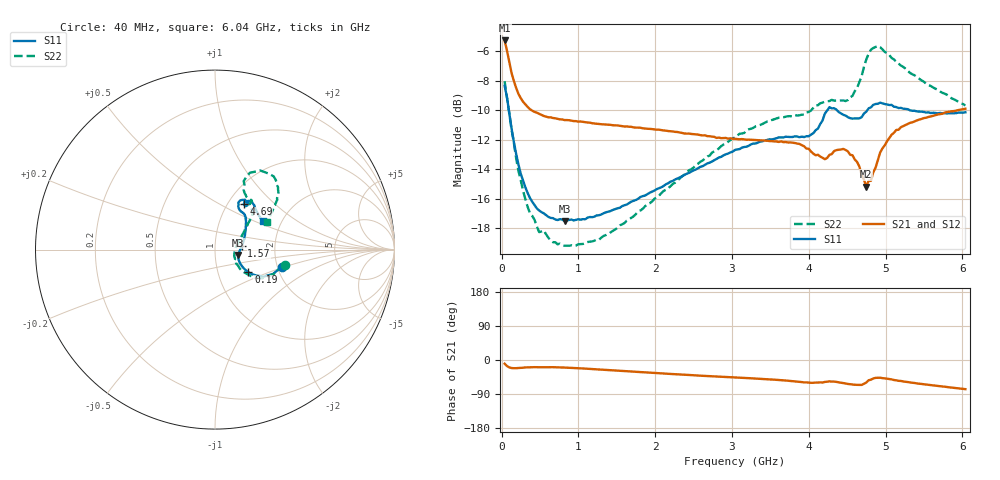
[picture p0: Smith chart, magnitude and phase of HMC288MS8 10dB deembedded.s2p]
!Hittite Microwave Corporation
!12 Elizabeth Drive
!Chelmsford, MA 01824
!Tel: 978-250-3343
!Fax: 978-250-3373
!Device: HMC288MS8, 0.7-3.7 GHz GaAs IC 3-bit Digital Attenuator in 8-lead Grounded Base surface Mount Plastic Package
!Misc:  10dB state, room
# GHZ S DB R 50.0
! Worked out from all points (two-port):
!   201 points, 40 MHz to 6.04 GHz, reference 50 ohm
!   highest |S21| = -5.26 dB at 40 MHz (marker M1); lowest = -15.2 dB at 4.75 GHz (marker M2)
!   |S21| within 3 dB of the highest: start of sweep to 176.5 MHz
!   lowest |S11| = -17.5 dB at 820 MHz (marker M3), VSWR 1.31, Z = 64.8 - j3.89 ohm
!   |S11| at or under -10 dB: 95.9 MHz to 4.242 GHz (4.146 GHz wide, 191 % of centre); 4.369 GHz to 4.762 GHz (392.4 MHz wide, 8.59 % of centre); 5.319 GHz to end of sweep
!   |S22| runs from -19.2 to -5.6 dB; largest |S21 - S12| = 0.0038
!   S11 on the Smith chart (normalised r, x): 40 MHz: 2.11, -0.47; 190 MHz: 1.40, -0.37; 1.57 GHz: 1.35, +0.05; 4.69 GHz: 1.18, +0.66; 6.04 GHz: 1.60, +0.57
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0.04  -8.33 -14.4  -5.26 -9.8  -5.32 -9.7  -8.02 -12.5
0.1  -10.14 -28.8  -6.70 -19.4  -6.74 -19.3  -10.22 -31.1
0.19  -12.94 -34.2  -8.48 -21.6  -8.49 -21.5  -13.25 -37.5
0.34  -15.61 -29.8  -9.77 -19.4  -9.76 -19.7  -16.54 -34.1
0.49  -16.79 -23.9  -10.24 -19.0  -10.22 -18.8  -18.25 -28.4
0.82  -17.49 -12.8  -10.66 -20.0  -10.63 -20.2  -19.18 -12.3
1.06  -17.38 -6.1  -10.78 -22.5  -10.77 -22.5  -19.06 -2.8
1.57  -16.50 7.3  -11.06 -28.8  -11.06 -28.9  -17.73 14.0
2.05  -15.28 20.1  -11.31 -34.9  -11.30 -35.0  -15.78 25.9
3.04  -12.69 41.6  -11.93 -46.0  -11.89 -46.1  -11.85 40.3
3.82  -11.76 52.6  -12.21 -56.2  -12.21 -56.2  -10.32 46.9
4.06  -11.55 60.0  -12.94 -60.2  -12.93 -60.2  -9.83 52.8
4.18  -10.69 63.6  -13.22 -59.4  -13.22 -59.6  -9.47 53.0
4.27  -9.79 59.0  -13.01 -56.4  -12.98 -56.6  -9.37 53.0
4.51  -10.46 54.4  -12.78 -63.2  -12.76 -63.5  -9.30 59.3
4.69  -10.46 57.7  -14.40 -65.8  -14.35 -66.0  -7.66 67.3
4.75  -10.09 58.4  -15.17 -59.4  -15.09 -59.1  -6.55 65.6
4.81  -9.80 56.5  -14.78 -51.9  -14.74 -52.3  -5.89 60.4
4.9  -9.56 53.5  -13.38 -46.8  -13.27 -46.4  -5.63 51.3
5.05  -9.64 48.9  -11.87 -50.4  -11.86 -50.7  -6.26 43.8
5.32  -10.00 43.7  -10.85 -59.3  -10.81 -59.4  -7.47 37.3
6.04  -10.13 31.3  -9.89 -76.9  -9.87 -77.0  -9.67 27.4
